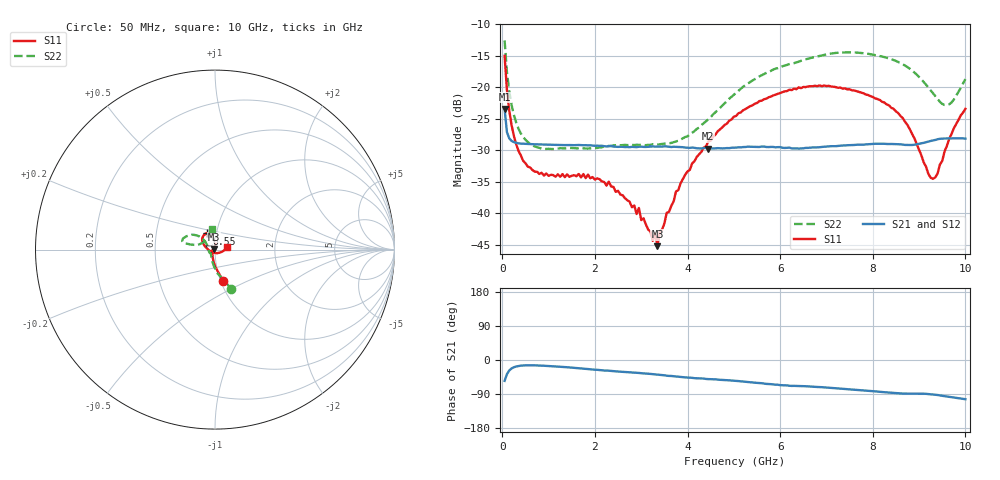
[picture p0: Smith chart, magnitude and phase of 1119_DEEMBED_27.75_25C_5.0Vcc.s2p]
!Hittite Microwave Corp.
!Digital Attenuator/PhaseShifter Rev 1.4.0
!Filename: C:\DATA\DATA\1119_DEEMBED_27.75_25C_5.0Vcc.s2p
!VNA ID: Agilent Technologies,N5224A,MY51441122,A.10.45.03
!Device type:
!2 Port Calibration.
!Temp(C): 25
!Lot Number:
!Serial Number:
!Operator:
!Misc:
!Attenuator:  27.750
# GHZ S DB R 50.0
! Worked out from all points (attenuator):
!   200 points, 50 MHz to 10 GHz, reference 50 ohm
!   highest |S21| = -23.43 dB at 50 MHz (marker M1); lowest = -29.7 dB at 4.45 GHz (marker M2)
!   lowest |S11| = -45.2 dB at 3.35 GHz (marker M3), VSWR 1.01, Z = 49.5 + j0.301 ohm
!   |S11| at or under -10 dB: start of sweep to end of sweep
!   |S22| runs from -29.8 to -12.6 dB; largest |S21 - S12| = 0.00013
!   S11 on the Smith chart (normalised r, x): 50 MHz: 1.03, -0.37; 6.55 GHz: 0.90, +0.16; 10 GHz: 1.14, +0.04
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0.05  -14.99 -75.7  -23.43 -55.1  -23.43 -55.1  -12.56 -67.4
0.1  -20.45 -89.3  -27.09 -37.4  -27.08 -37.4  -17.51 -83.9
0.2  -25.97 -103.6  -28.49 -22.3  -28.49 -22.3  -22.79 -100.5
0.45  -31.65 -125.2  -28.94 -14.4  -28.94 -14.4  -27.88 -121.3
0.9  -34.00 -146.0  -29.07 -15.2  -29.07 -15.2  -29.76 -135.8
1.75  -33.75 -153.7  -29.18 -22.8  -29.17 -22.8  -29.67 -140.8
2.3  -34.96 -156.6  -29.32 -28.4  -29.32 -28.4  -29.29 -149.2
2.95  -39.13 -151.1  -29.42 -34.2  -29.42 -34.2  -29.12 -160.1
3.25  -44.35 173.6  -29.37 -37.6  -29.38 -37.6  -29.01 -168.8
3.3  -43.11 162.3  -29.40 -38.2  -29.40 -38.3  -29.05 -170.5
3.35  -45.19 146.5  -29.40 -38.8  -29.41 -38.8  -29.09 -172.2
3.4  -42.85 145.6  -29.39 -39.1  -29.40 -39.2  -29.03 -173.6
3.75  -36.53 99.5  -29.44 -43.6  -29.44 -43.6  -28.57 173.2
4.45  -28.57 85.0  -29.71 -50.4  -29.72 -50.4  -25.05 146.2
5.05  -24.53 92.3  -29.55 -55.0  -29.56 -55.1  -20.83 138.7
6.55  -19.96 116.3  -29.60 -69.2  -29.61 -69.3  -15.56 152.2
6.7  -19.82 120.0  -29.53 -70.4  -29.55 -70.4  -15.25 153.9
8.35  -22.85 153.8  -28.99 -85.9  -28.99 -85.9  -15.41 168.1
8.75  -25.98 167.9  -29.14 -88.7  -29.13 -88.7  -16.79 168.1
9.3  -34.51 -99.6  -28.42 -91.0  -28.43 -91.0  -20.92 160.1
9.65  -28.18 -19.8  -28.09 -97.2  -28.10 -97.2  -22.68 126.1
10  -23.40 13.6  -28.13 -103.5  -28.13 -103.5  -18.69 98.4
